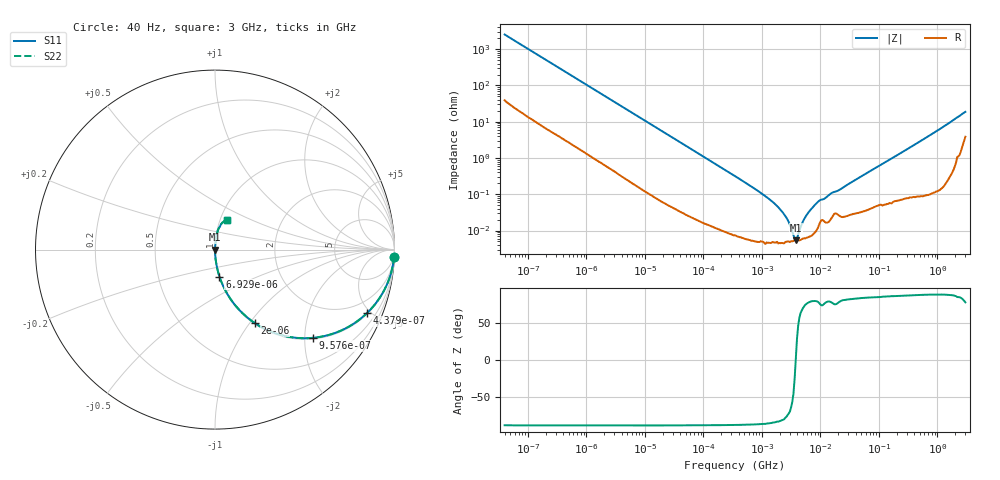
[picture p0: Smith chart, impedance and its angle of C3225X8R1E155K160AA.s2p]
! S-parameter Generated by TDK Corporation
! Copyright(C) 2015 TDK Corporation.
! All Rights Reserved.
! TDK P/N: C3225X8R1E155K160AA (Multilayer Ceramic Chip Capacitors)
! Property: C=1.5uF
! Size(LxWxT): 3.2x2.5x1.6mm, 0.126x0.098x0.063inches
! Model Type: s2p (Touchstone File Format Version 1.0)
! Frequency: DC=Yes Start=0.00004MHz Stop=3000MHz 396points Log-sweep
! Note: This model was converted from impedance.
! Model Generated on Jun. 23, 2015
! Hash(MD5):
! Port Assignments:
!  1 ---| |--- 2
! Applicable Conditions:
!  Temperature = 25 degC
!  DC Bias Voltage = 0 V
!  Small Signal Operation
! Terms and conditions regarding TDK Simulation Models
! (1)This simulation model is being provided solely for informational purposes. Please refer to the specifications of the products in terms of detailed characteristics of such products.
! (2)In no event shall TDK Corporation of any of its subsidiaries be liable for any loss or damage arising, directly or indirectly,
!  From any information contained in this simulation model, including, but not limited to loss or damages arising from any inaccuracies, omissions or errors in connection with such information.
! (3)Any and all copyrights on this simulation model are owned by TDK Corporation.
!  Duplication or redistribution of this simulation model without prior written permission from TDK Corporation is prohibited.
! (4)This simulation model is subject to any modification or change without any prior notice.
! (5)Neither TDK Corporation nor any of its subsidiaries shall make any warranty, express or implied,
!  Including but not limited to the correctness, implied warranties of merchantability and fitness for a particular purpose with respect to this simulation models.
! (6)The use of this simulation model shall be deemed to have consented to the terms and conditions hereof.
# MHz S MA R 50
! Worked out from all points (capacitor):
!   395 points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, 40 Hz to 3 GHz, reference 50 ohm
!   read as one part in series: C = 1.57 uF near 41.88 Hz
!   lowest |Z| = 5.42 mohm at 3.793 MHz (marker M1)
!   series resonance near 3.785 MHz, so ESL is about 1.1 nH
!   S11 on the Smith chart (normalised r, x): 40 Hz: 2, -51; 437.9 Hz: 1.06, -4.75; 957.6 Hz: 1.03, -2.19; 2 kHz: 1.01, -1.06; 6.929 kHz: 1.00, -0.31; 3 GHz: 1.08, +0.37
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4e-05  0.9986 -2.2  0.03922 86.9  0.03922 86.9  0.9986 -2.2
0.0001451139  0.9884 -8.0  0.1394 81.2  0.1394 81.2  0.9884 -8.0
0.0002763971  0.9632 -14.9  0.2569 74.4  0.2569 74.4  0.9632 -14.9
0.0004379335  0.9176 -22.7  0.386 66.6  0.386 66.6  0.9176 -22.7
0.000834128  0.7773 -38.3  0.6193 51.0  0.6193 51.0  0.7773 -38.3
0.0009576241  0.7338 -42.1  0.6702 47.2  0.6702 47.2  0.7338 -42.1
0.001999837  0.4646 -61.6  0.8799 27.7  0.8799 27.7  0.4646 -61.6
0.003474114  0.2914 -72.4  0.9531 16.9  0.9531 16.9  0.2914 -72.4
0.006928769  0.1524 -80.6  0.9866 8.8  0.9866 8.8  0.1524 -80.6
0.01739424  0.06191 -85.8  0.9974 3.5  0.9974 3.5  0.06191 -85.8
0.3464102  0.003172 -88.5  0.9999 0.2  0.9999 0.2  0.003172 -88.5
1.581893  0.000586 -85.3  1 0.0  1 0.0  0.000586 -85.3
2.506407  0.0002535 -78.9  1 0.0  1 0.0  0.0002535 -78.9
3.303516  9.361e-05 -57.2  0.9999 0.0  0.9999 0.0  9.361e-05 -57.2
3.792615  5.42e-05 1.3  0.9999 -0.0  0.9999 -0.0  5.42e-05 1.3
4.354128  9.833e-05 56.8  0.9999 -0.0  0.9999 -0.0  9.833e-05 56.8
5.234209  0.0002036 72.5  0.9999 -0.0  0.9999 -0.0  0.0002036 72.5
7.22376  0.0004197 79.8  0.9999 -0.0  0.9999 -0.0  0.0004197 79.8
9.521122  0.0006644 77.2  0.9999 -0.0  0.9999 -0.0  0.0006644 77.2
150.6385  0.008884 85.8  0.9994 -0.5  0.9994 -0.5  0.008884 85.8
906.6656  0.05169 85.8  0.9975 -3.0  0.9975 -3.0  0.05169 85.8
3000  0.1776 68.1  0.9482 -10.0  0.9482 -10.0  0.1776 68.1
